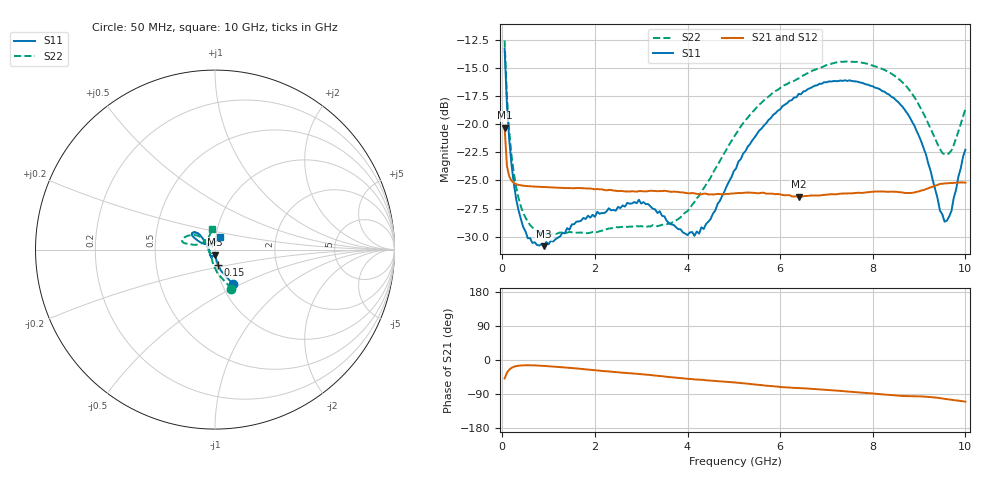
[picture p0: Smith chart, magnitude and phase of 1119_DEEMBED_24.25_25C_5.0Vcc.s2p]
!Hittite Microwave Corp.
!Digital Attenuator/PhaseShifter Rev 1.4.0
!Filename: C:\DATA\DATA\1119_DEEMBED_24.25_25C_5.0Vcc.s2p
!VNA ID: Agilent Technologies,N5224A,MY51441122,A.10.45.03
!Device type:
!2 Port Calibration.
!Temp(C): 25
!Lot Number:
!Serial Number:
!Operator:
!Misc:
!Attenuator:  24.250
# GHZ S DB R 50.0
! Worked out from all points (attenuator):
!   200 points, 50 MHz to 10 GHz, reference 50 ohm
!   highest |S21| = -20.31 dB at 50 MHz (marker M1); lowest = -26.4 dB at 6.4 GHz (marker M2)
!   lowest |S11| = -30.9 dB at 900 MHz (marker M3), VSWR 1.06, Z = 49.7 - j2.84 ohm
!   |S11| at or under -10 dB: start of sweep to end of sweep
!   |S22| runs from -29.8 to -12.6 dB; largest |S21 - S12| = 0.00017
!   S11 on the Smith chart (normalised r, x): 50 MHz: 1.13, -0.45; 150 MHz: 1.02, -0.17; 10 GHz: 1.05, +0.15
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0.05  -13.29 -62.5  -20.31 -48.6  -20.31 -48.6  -12.55 -67.2
0.1  -18.25 -74.2  -23.70 -33.9  -23.70 -33.9  -17.51 -83.8
0.15  -21.36 -79.0  -24.66 -25.4  -24.66 -25.4  -20.64 -93.4
0.3  -26.67 -84.4  -25.33 -16.2  -25.33 -16.2  -25.59 -110.5
0.45  -29.13 -86.0  -25.47 -14.1  -25.47 -14.0  -27.87 -121.2
0.65  -30.56 -90.8  -25.54 -14.0  -25.53 -14.1  -29.18 -130.0
0.9  -30.85 -94.5  -25.59 -15.6  -25.59 -15.6  -29.76 -135.6
1.75  -28.34 -110.4  -25.70 -24.1  -25.70 -24.1  -29.65 -140.5
2.95  -26.72 -119.4  -25.95 -36.8  -25.96 -36.8  -29.09 -159.8
3.4  -27.75 -132.4  -25.95 -42.1  -25.95 -42.1  -29.01 -173.3
3.9  -29.63 -156.3  -26.06 -48.4  -26.07 -48.5  -28.07 167.0
4.25  -29.73 -178.5  -26.22 -52.0  -26.23 -52.1  -26.37 152.5
5.05  -23.92 143.0  -26.14 -59.6  -26.16 -59.6  -20.83 138.9
5.55  -20.56 137.2  -26.14 -65.6  -26.15 -65.7  -18.26 141.3
6.4  -17.30 137.0  -26.45 -74.0  -26.47 -74.1  -15.92 150.0
6.7  -16.68 139.3  -26.34 -76.3  -26.35 -76.2  -15.23 154.0
7.5  -16.10 145.8  -26.15 -83.6  -26.16 -83.6  -14.43 163.6
8.35  -17.35 150.1  -26.01 -92.1  -26.01 -92.1  -15.38 168.1
8.999999  -21.07 153.6  -25.97 -96.0  -25.98 -96.0  -18.31 167.3
9.55  -28.67 115.9  -25.27 -102.5  -25.28 -102.5  -22.69 138.1
9.7  -27.70 88.2  -25.23 -104.8  -25.24 -104.8  -22.32 120.0
10  -22.27 67.1  -25.20 -109.8  -25.20 -109.8  -18.63 98.5
